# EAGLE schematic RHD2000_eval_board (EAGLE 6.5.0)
RHD2000 Evaluation Board

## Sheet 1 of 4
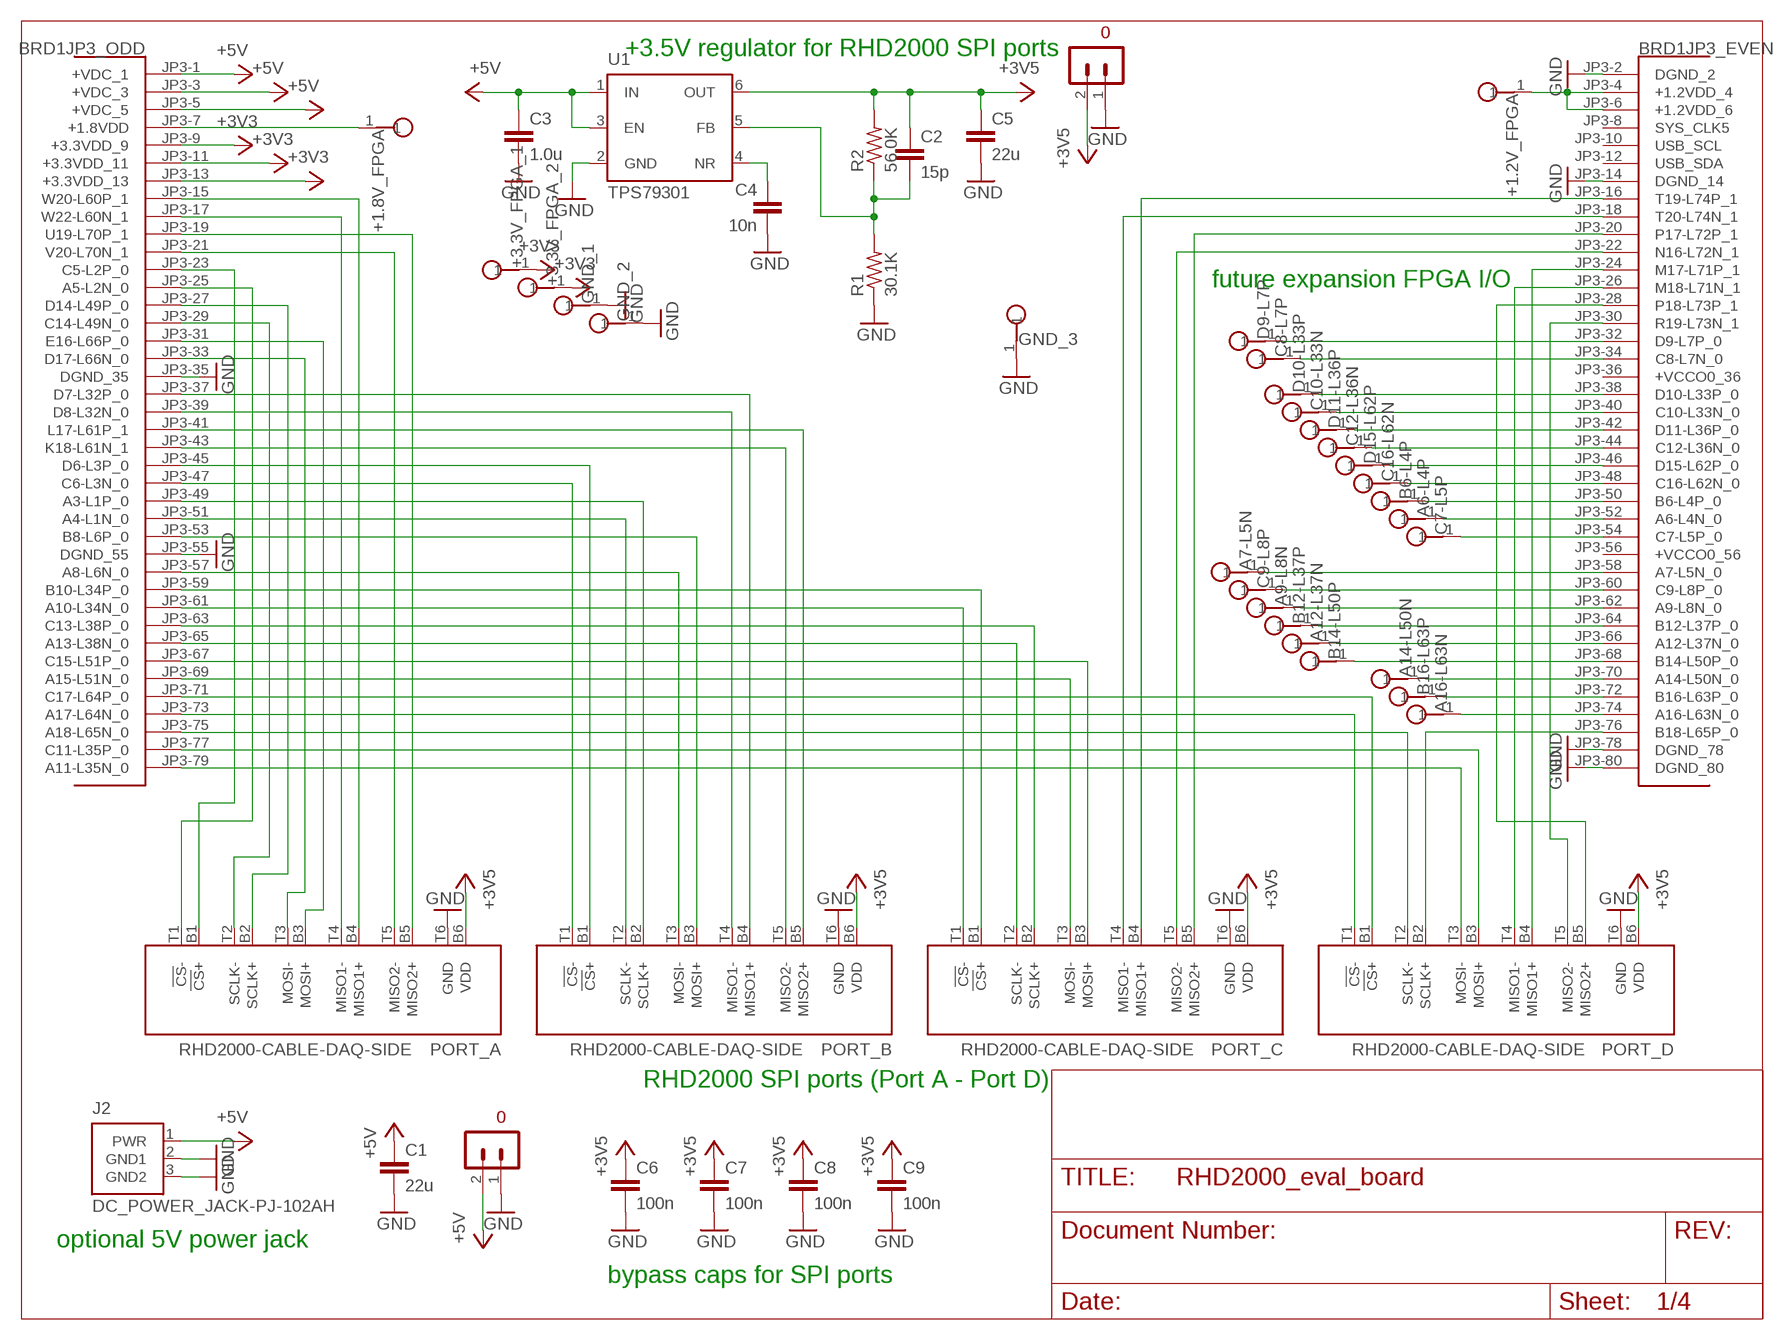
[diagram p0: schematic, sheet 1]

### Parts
+1.2V_FPGA  TESTPOINT  [TESTPOINT]
+1.8V_FPGA  TESTPOINT  [TESTPOINT]
+3.3V_FPGA_1  TESTPOINT  [TESTPOINT]
+3.3V_FPGA_2  TESTPOINT  [TESTPOINT]
A6-L4P  TESTPOINT  [TESTPOINT]
A7-L5N  TESTPOINT  [TESTPOINT]
A9-L8N  TESTPOINT  [TESTPOINT]
A12-L37N  TESTPOINT  [TESTPOINT]
A14-L50N  TESTPOINT  [TESTPOINT]
A16-L63N  TESTPOINT  [TESTPOINT]
B6-L4P  TESTPOINT  [TESTPOINT]
B12-L37P  TESTPOINT  [TESTPOINT]
B14-L50P  TESTPOINT  [TESTPOINT]
B16-L63P  TESTPOINT  [TESTPOINT]
BRD1  OPALKELLY_XEM6010  [OPALKELLY_XEM6010]
C1  22u  C_1206  [1206]
C2  15p  C_0603  [0603]
C3  1.0u  C_0805  [0805]
C4  10n  C_0603  [0603]
C5  22u  C_1206  [1206]
C6  100n  C_0603  [0603]
C7  100n  C_0603  [0603]
C7-L5P  TESTPOINT  [TESTPOINT]
C8  100n  C_0603  [0603]
C8-L7P  TESTPOINT  [TESTPOINT]
C9  100n  C_0603  [0603]
C9-L8P  TESTPOINT  [TESTPOINT]
C10-L33N  TESTPOINT  [TESTPOINT]
C12-L36N  TESTPOINT  [TESTPOINT]
C16-L62N  TESTPOINT  [TESTPOINT]
D9-L7P  TESTPOINT  [TESTPOINT]
D10-L33P  TESTPOINT  [TESTPOINT]
D11-L36P  TESTPOINT  [TESTPOINT]
D15-L62P  TESTPOINT  [TESTPOINT]
GND_1  TESTPOINT  [TESTPOINT]
GND_2  TESTPOINT  [TESTPOINT]
GND_3  TESTPOINT  [TESTPOINT]
J2  DC_POWER_JACK-PJ-102AH  [PJ-102AH]
PORT_A  RHD2000-CABLE-DAQ-SIDE  [OMNETICS_PZN-12-AA]
PORT_B  RHD2000-CABLE-DAQ-SIDE  [OMNETICS_PZN-12-AA]
PORT_C  RHD2000-CABLE-DAQ-SIDE  [OMNETICS_PZN-12-AA]
PORT_D  RHD2000-CABLE-DAQ-SIDE  [OMNETICS_PZN-12-AA]
R1  30.1K  R_0603  [0603]
R2  56.0K  R_0603  [0603]
S9  TERMINAL_BLOCK_2-3.5MM-5V  [TERMINAL_BLOCK_3.5MM_2_5V]
S10  TERMINAL_BLOCK_2-3.5MM-3.5V  [TERMINAL_BLOCK_3.5MM_2_3.5V]
U1  TPS79301  [SOT-23-6]

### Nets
+3V3 [power]: +3.3V_FPGA_1.1 +3.3V_FPGA_2.1 BRD1.JP3-9(JP3_ODD:+3.3VDD_9) BRD1.JP3-11(JP3_ODD:+3.3VDD_11) BRD1.JP3-13(JP3_ODD:+3.3VDD_13) ; also sheet 3
+3V5 [power]: C2.1 C5.1 C6.1 C7.1 C8.1 C9.1 PORT_A.B6(VDD) PORT_B.B6(VDD) PORT_C.B6(VDD) PORT_D.B6(VDD) R2.2 S10.2 U1.6(OUT)
+5V [power]: BRD1.JP3-1(JP3_ODD:+VDC_1) BRD1.JP3-3(JP3_ODD:+VDC_3) BRD1.JP3-5(JP3_ODD:+VDC_5) C1.1 C3.1 J2.1(PWR) S9.2 U1.1(IN) U1.3(EN) ; also sheet 2,4
GND [power]: BRD1.JP3-2(JP3_EVEN:DGND_2) BRD1.JP3-14(JP3_EVEN:DGND_14) BRD1.JP3-35(JP3_ODD:DGND_35) BRD1.JP3-55(JP3_ODD:DGND_55) BRD1.JP3-78(JP3_EVEN:DGND_78) BRD1.JP3-80(JP3_EVEN:DGND_80) C1.2 C3.2 C4.2 C5.2 C6.2 C7.2 C8.2 C9.2 GND_1.1 GND_2.1 GND_3.1 J2.2(GND1) J2.3(GND2) PORT_A.T6(GND) PORT_B.T6(GND) PORT_C.T6(GND) PORT_D.T6(GND) R1.1 S9.1 S10.1 U1.2(GND) ; also sheet 2,3,4
N$1: BRD1.JP3-15(JP3_ODD:W20-L60P_1) PORT_A.B4(MISO1+)
N$2: BRD1.JP3-17(JP3_ODD:W22-L60N_1) PORT_A.T4(MISO1-)
N$3: BRD1.JP3-19(JP3_ODD:U19-L70P_1) PORT_A.B5(MISO2+)
N$4: BRD1.JP3-21(JP3_ODD:V20-L70N_1) PORT_A.T5(MISO2-)
N$5: BRD1.JP3-23(JP3_ODD:C5-L2P_0) PORT_A.B1(!CS!+)
N$6: BRD1.JP3-25(JP3_ODD:A5-L2N_0) PORT_A.T1(!CS!-)
N$7: BRD1.JP3-27(JP3_ODD:D14-L49P_0) PORT_A.B2(SCLK+)
N$8: BRD1.JP3-29(JP3_ODD:C14-L49N_0) PORT_A.T2(SCLK-)
N$9: BRD1.JP3-31(JP3_ODD:E16-L66P_0) PORT_A.B3(MOSI+)
N$10: BRD1.JP3-33(JP3_ODD:D17-L66N_0) PORT_A.T3(MOSI-)
N$11: BRD1.JP3-37(JP3_ODD:D7-L32P_0) PORT_B.B4(MISO1+)
N$12: BRD1.JP3-39(JP3_ODD:D8-L32N_0) PORT_B.T4(MISO1-)
N$13: BRD1.JP3-41(JP3_ODD:L17-L61P_1) PORT_B.B5(MISO2+)
N$14: BRD1.JP3-43(JP3_ODD:K18-L61N_1) PORT_B.T5(MISO2-)
N$15: BRD1.JP3-45(JP3_ODD:D6-L3P_0) PORT_B.B1(!CS!+)
N$16: BRD1.JP3-47(JP3_ODD:C6-L3N_0) PORT_B.T1(!CS!-)
N$17: BRD1.JP3-49(JP3_ODD:A3-L1P_0) PORT_B.B2(SCLK+)
N$18: BRD1.JP3-51(JP3_ODD:A4-L1N_0) PORT_B.T2(SCLK-)
N$19: BRD1.JP3-53(JP3_ODD:B8-L6P_0) PORT_B.B3(MOSI+)
N$20: BRD1.JP3-57(JP3_ODD:A8-L6N_0) PORT_B.T3(MOSI-)
N$21: BRD1.JP3-59(JP3_ODD:B10-L34P_0) PORT_C.B1(!CS!+)
N$22: BRD1.JP3-61(JP3_ODD:A10-L34N_0) PORT_C.T1(!CS!-)
N$23: BRD1.JP3-63(JP3_ODD:C13-L38P_0) PORT_C.B2(SCLK+)
N$24: BRD1.JP3-65(JP3_ODD:A13-L38N_0) PORT_C.T2(SCLK-)
N$25: BRD1.JP3-67(JP3_ODD:C15-L51P_0) PORT_C.B3(MOSI+)
N$26: BRD1.JP3-69(JP3_ODD:A15-L51N_0) PORT_C.T3(MOSI-)
N$27: BRD1.JP3-71(JP3_ODD:C17-L64P_0) PORT_D.B1(!CS!+)
N$28: BRD1.JP3-73(JP3_ODD:A17-L64N_0) PORT_D.T1(!CS!-)
N$29: BRD1.JP3-75(JP3_ODD:A18-L65N_0) PORT_D.T2(SCLK-)
N$30: BRD1.JP3-77(JP3_ODD:C11-L35P_0) PORT_D.B3(MOSI+)
N$31: BRD1.JP3-79(JP3_ODD:A11-L35N_0) PORT_D.T3(MOSI-)
N$32: BRD1.JP3-76(JP3_EVEN:B18-L65P_0) PORT_D.B2(SCLK+)
N$33: BRD1.JP3-16(JP3_EVEN:T19-L74P_1) PORT_C.B4(MISO1+)
N$34: BRD1.JP3-18(JP3_EVEN:T20-L74N_1) PORT_C.T4(MISO1-)
N$35: BRD1.JP3-20(JP3_EVEN:P17-L72P_1) PORT_C.B5(MISO2+)
N$36: BRD1.JP3-22(JP3_EVEN:N16-L72N_1) PORT_C.T5(MISO2-)
N$37: BRD1.JP3-24(JP3_EVEN:M17-L71P_1) PORT_D.B4(MISO1+)
N$38: BRD1.JP3-26(JP3_EVEN:M18-L71N_1) PORT_D.T4(MISO1-)
N$39: BRD1.JP3-28(JP3_EVEN:P18-L73P_1) PORT_D.B5(MISO2+)
N$40: BRD1.JP3-30(JP3_EVEN:R19-L73N_1) PORT_D.T5(MISO2-)
N$143: C4.1 U1.4(NR)
N$144: C2.2 R1.2 R2.1 U1.5(FB)
N$173: BRD1.JP3-32(JP3_EVEN:D9-L7P_0) D9-L7P.1
N$174: BRD1.JP3-34(JP3_EVEN:C8-L7N_0) C8-L7P.1
N$175 [power]: +1.8V_FPGA.1 BRD1.JP3-7(JP3_ODD:+1.8VDD)
N$176: BRD1.JP3-38(JP3_EVEN:D10-L33P_0) D10-L33P.1
N$177: BRD1.JP3-40(JP3_EVEN:C10-L33N_0) C10-L33N.1
N$178: BRD1.JP3-42(JP3_EVEN:D11-L36P_0) D11-L36P.1
N$179: BRD1.JP3-44(JP3_EVEN:C12-L36N_0) C12-L36N.1
N$180: BRD1.JP3-46(JP3_EVEN:D15-L62P_0) D15-L62P.1
N$181: BRD1.JP3-48(JP3_EVEN:C16-L62N_0) C16-L62N.1
N$182: B6-L4P.1 BRD1.JP3-50(JP3_EVEN:B6-L4P_0)
N$183: A6-L4P.1 BRD1.JP3-52(JP3_EVEN:A6-L4N_0)
N$184: BRD1.JP3-54(JP3_EVEN:C7-L5P_0) C7-L5P.1
N$185 [power]: +1.2V_FPGA.1 BRD1.JP3-4(JP3_EVEN:+1.2VDD_4) BRD1.JP3-6(JP3_EVEN:+1.2VDD_6)
N$186: A7-L5N.1 BRD1.JP3-58(JP3_EVEN:A7-L5N_0)
N$187: BRD1.JP3-60(JP3_EVEN:C9-L8P_0) C9-L8P.1
N$188: A9-L8N.1 BRD1.JP3-62(JP3_EVEN:A9-L8N_0)
N$189: B12-L37P.1 BRD1.JP3-64(JP3_EVEN:B12-L37P_0)
N$190: A12-L37N.1 BRD1.JP3-66(JP3_EVEN:A12-L37N_0)
N$191: B14-L50P.1 BRD1.JP3-68(JP3_EVEN:B14-L50P_0)
N$192: A14-L50N.1 BRD1.JP3-70(JP3_EVEN:A14-L50N_0)
N$193: B16-L63P.1 BRD1.JP3-72(JP3_EVEN:B16-L63P_0)
N$194: A16-L63N.1 BRD1.JP3-74(JP3_EVEN:A16-L63N_0)
Unconnected: BRD1.JP3-8(JP3_EVEN:SYS_CLK5) BRD1.JP3-10(JP3_EVEN:USB_SCL) BRD1.JP3-12(JP3_EVEN:USB_SDA)

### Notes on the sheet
- +3.5V regulator for RHD2000 SPI ports
- future expansion FPGA I/O
- RHD2000 SPI ports (Port A - Port D)
- optional 5V power jack
- bypass caps for SPI ports

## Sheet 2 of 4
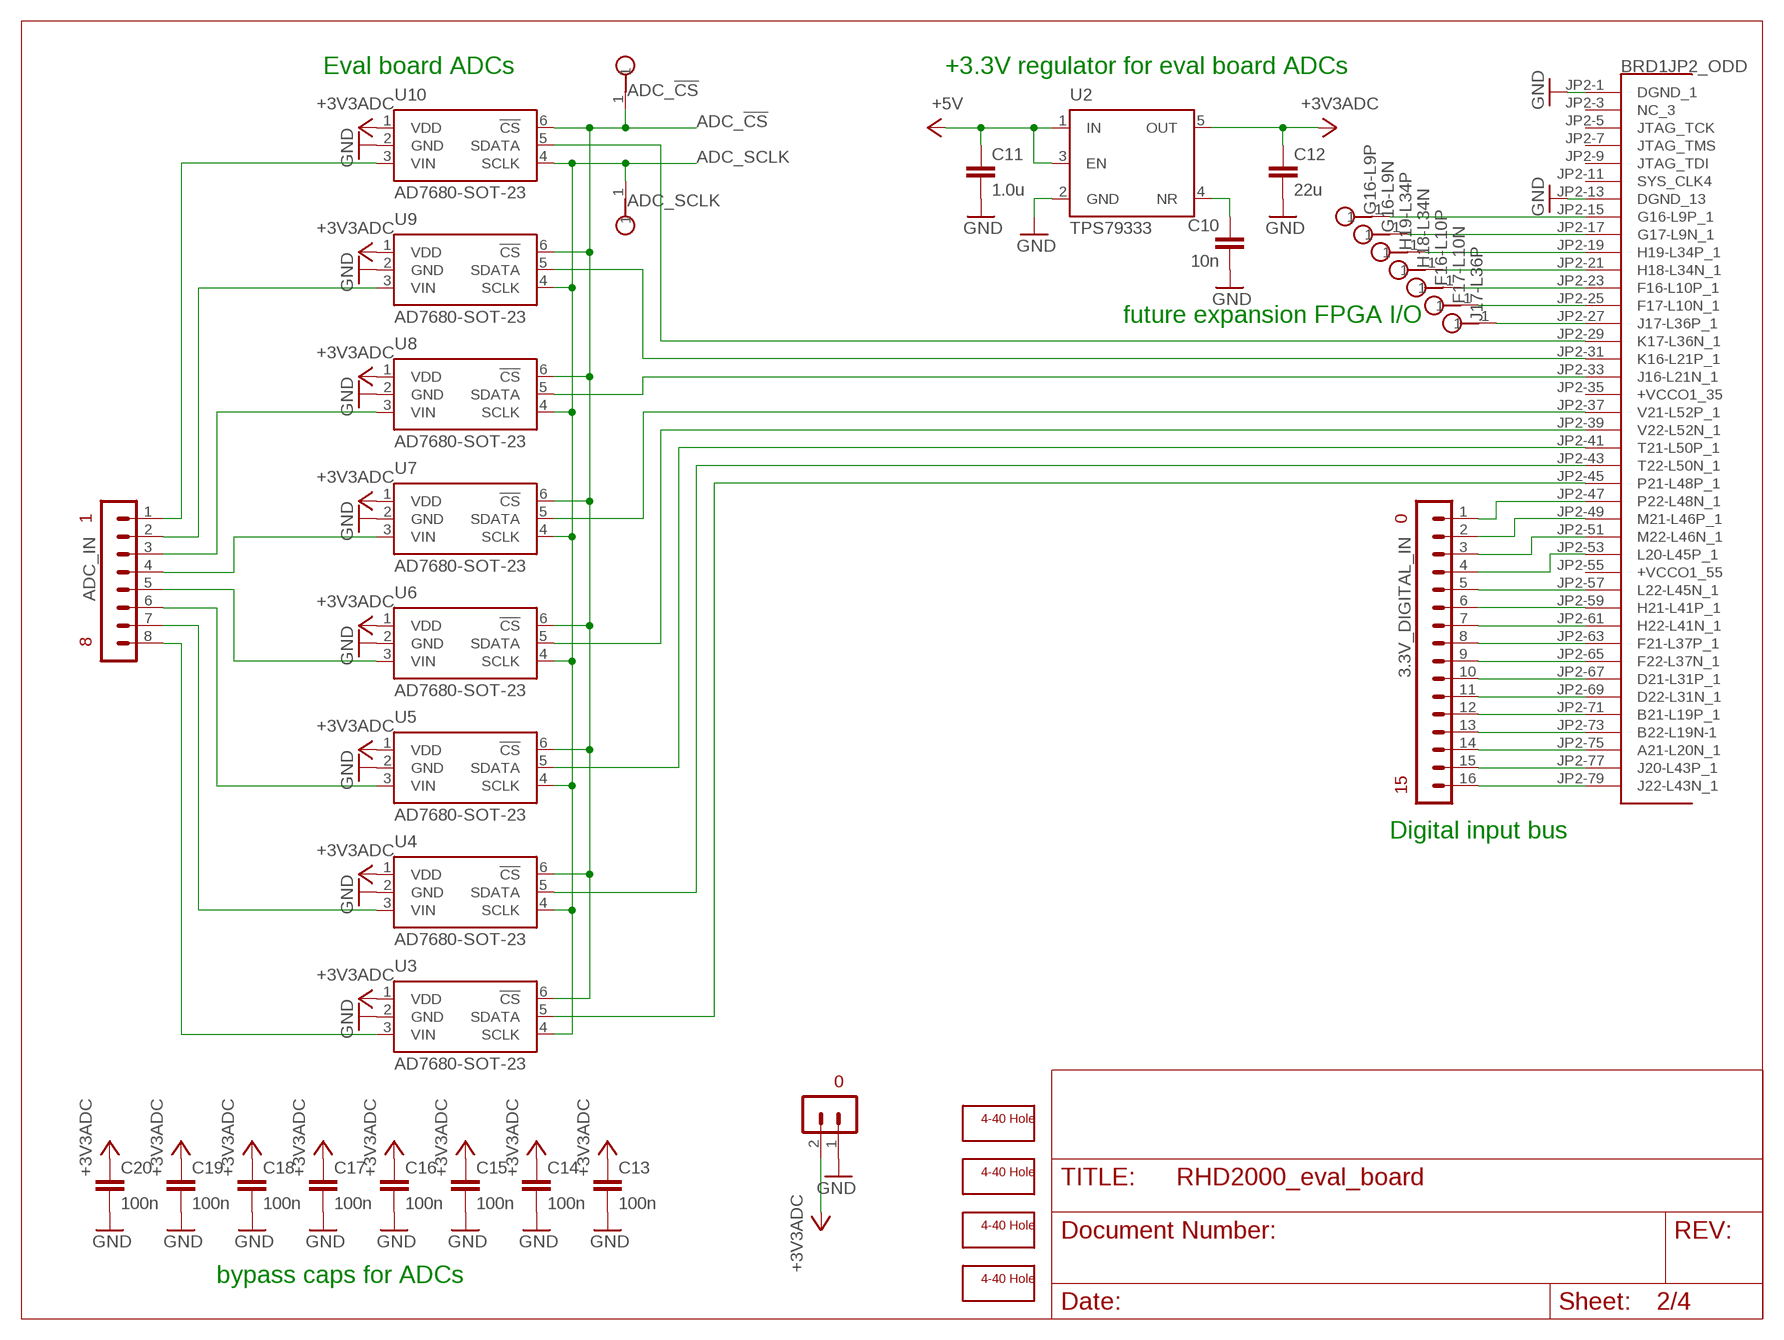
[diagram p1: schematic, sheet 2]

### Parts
3.3V_DIGITAL_IN  TERMINAL_BLOCK_16-3.5MM  [TERMINAL_BLOCK_3.5MM_16]
ADC_!CS!  TESTPOINT  [TESTPOINT]
ADC_IN  TERMINAL_BLOCK_8-3.5MM  [TERMINAL_BLOCK_3.5MM_8]
ADC_SCLK  TESTPOINT  [TESTPOINT]
C10  10n  C_0603  [0603]
C11  1.0u  C_0805  [0805]
C12  22u  C_1206  [1206]
C13  100n  C_0603  [0603]
C14  100n  C_0603  [0603]
C15  100n  C_0603  [0603]
C16  100n  C_0603  [0603]
C17  100n  C_0603  [0603]
C18  100n  C_0603  [0603]
C19  100n  C_0603  [0603]
C20  100n  C_0603  [0603]
F16-L10P  TESTPOINT  [TESTPOINT]
F17-L10N  TESTPOINT  [TESTPOINT]
G16-L9N  TESTPOINT  [TESTPOINT]
G16-L9P  TESTPOINT  [TESTPOINT]
H1  SCREW_HOLE_4-40  [SCREW_HOLE_4-40]
H2  SCREW_HOLE_4-40  [SCREW_HOLE_4-40]
H3  SCREW_HOLE_4-40  [SCREW_HOLE_4-40]
H4  SCREW_HOLE_4-40  [SCREW_HOLE_4-40]
H18-L34N  TESTPOINT  [TESTPOINT]
H19-L34P  TESTPOINT  [TESTPOINT]
J17-L36P  TESTPOINT  [TESTPOINT]
S2  TERMINAL_BLOCK_2-3.5MM-3.3V  [TERMINAL_BLOCK_3.5MM_2_3.3V]
U2  TPS79333  [SOT-23-5]
U3  AD7680-SOT-23  [SOT-23-RJ-6]
U4  AD7680-SOT-23  [SOT-23-RJ-6]
U5  AD7680-SOT-23  [SOT-23-RJ-6]
U6  AD7680-SOT-23  [SOT-23-RJ-6]
U7  AD7680-SOT-23  [SOT-23-RJ-6]
U8  AD7680-SOT-23  [SOT-23-RJ-6]
U9  AD7680-SOT-23  [SOT-23-RJ-6]
U10  AD7680-SOT-23  [SOT-23-RJ-6]

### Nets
+3V3ADC [power]: C12.1 C13.1 C14.1 C15.1 C16.1 C17.1 C18.1 C19.1 C20.1 S2.2 U2.5(OUT) U3.1(VDD) U4.1(VDD) U5.1(VDD) U6.1(VDD) U7.1(VDD) U8.1(VDD) U9.1(VDD) U10.1(VDD)
+5V [power]: C11.1 U2.1(IN) U2.3(EN) ; also sheet 1,4
ADC_!CS!: ADC_!CS!.1 U3.6(!CS!) U4.6(!CS!) U5.6(!CS!) U6.6(!CS!) U7.6(!CS!) U8.6(!CS!) U9.6(!CS!) U10.6(!CS!) ; also sheet 3
ADC_SCLK: ADC_SCLK.1 U3.4(SCLK) U4.4(SCLK) U5.4(SCLK) U6.4(SCLK) U7.4(SCLK) U8.4(SCLK) U9.4(SCLK) U10.4(SCLK) ; also sheet 3
GND [power]: BRD1.JP2-1(JP2_ODD:DGND_1) BRD1.JP2-13(JP2_ODD:DGND_13) C10.2 C11.2 C12.2 C13.2 C14.2 C15.2 C16.2 C17.2 C18.2 C19.2 C20.2 S2.1 U2.2(GND) U3.2(GND) U4.2(GND) U5.2(GND) U6.2(GND) U7.2(GND) U8.2(GND) U9.2(GND) U10.2(GND) ; also sheet 1,3,4
N$52: BRD1.JP2-29(JP2_ODD:K17-L36N_1) U10.5(SDATA)
N$54: BRD1.JP2-43(JP2_ODD:T22-L50N_1) U4.5(SDATA)
N$55: BRD1.JP2-31(JP2_ODD:K16-L21P_1) U9.5(SDATA)
N$56: BRD1.JP2-33(JP2_ODD:J16-L21N_1) U8.5(SDATA)
N$57: BRD1.JP2-37(JP2_ODD:V21-L52P_1) U7.5(SDATA)
N$58: BRD1.JP2-39(JP2_ODD:V22-L52N_1) U6.5(SDATA)
N$59: BRD1.JP2-41(JP2_ODD:T21-L50P_1) U5.5(SDATA)
N$60: BRD1.JP2-45(JP2_ODD:P21-L48P_1) U3.5(SDATA)
N$68: 3.3V_DIGITAL_IN.16 BRD1.JP2-79(JP2_ODD:J22-L43N_1)
N$69: 3.3V_DIGITAL_IN.15 BRD1.JP2-77(JP2_ODD:J20-L43P_1)
N$70: 3.3V_DIGITAL_IN.14 BRD1.JP2-75(JP2_ODD:A21-L20N_1)
N$71: 3.3V_DIGITAL_IN.13 BRD1.JP2-73(JP2_ODD:B22-L19N-1)
N$72: 3.3V_DIGITAL_IN.12 BRD1.JP2-71(JP2_ODD:B21-L19P_1)
N$73: 3.3V_DIGITAL_IN.11 BRD1.JP2-69(JP2_ODD:D22-L31N_1)
N$74: 3.3V_DIGITAL_IN.10 BRD1.JP2-67(JP2_ODD:D21-L31P_1)
N$75: 3.3V_DIGITAL_IN.9 BRD1.JP2-65(JP2_ODD:F22-L37N_1)
N$76: 3.3V_DIGITAL_IN.8 BRD1.JP2-63(JP2_ODD:F21-L37P_1)
N$77: 3.3V_DIGITAL_IN.7 BRD1.JP2-61(JP2_ODD:H22-L41N_1)
N$78: 3.3V_DIGITAL_IN.6 BRD1.JP2-59(JP2_ODD:H21-L41P_1)
N$79: 3.3V_DIGITAL_IN.5 BRD1.JP2-57(JP2_ODD:L22-L45N_1)
N$80: 3.3V_DIGITAL_IN.4 BRD1.JP2-53(JP2_ODD:L20-L45P_1)
N$81: 3.3V_DIGITAL_IN.3 BRD1.JP2-51(JP2_ODD:M22-L46N_1)
N$82: 3.3V_DIGITAL_IN.2 BRD1.JP2-49(JP2_ODD:M21-L46P_1)
N$83: 3.3V_DIGITAL_IN.1 BRD1.JP2-47(JP2_ODD:P22-L48N_1)
N$100: ADC_IN.1 U10.3(VIN)
N$101: ADC_IN.2 U9.3(VIN)
N$102: ADC_IN.3 U8.3(VIN)
N$103: ADC_IN.4 U7.3(VIN)
N$104: ADC_IN.5 U6.3(VIN)
N$105: ADC_IN.6 U5.3(VIN)
N$106: ADC_IN.7 U4.3(VIN)
N$107: ADC_IN.8 U3.3(VIN)
N$108: C10.1 U2.4(NR)
N$165: BRD1.JP2-15(JP2_ODD:G16-L9P_1) G16-L9P.1
N$166: BRD1.JP2-17(JP2_ODD:G17-L9N_1) G16-L9N.1
N$167: BRD1.JP2-19(JP2_ODD:H19-L34P_1) H19-L34P.1
N$168: BRD1.JP2-21(JP2_ODD:H18-L34N_1) H18-L34N.1
N$169: BRD1.JP2-23(JP2_ODD:F16-L10P_1) F16-L10P.1
N$170: BRD1.JP2-25(JP2_ODD:F17-L10N_1) F17-L10N.1
N$171: BRD1.JP2-27(JP2_ODD:J17-L36P_1) J17-L36P.1
Unconnected: BRD1.JP2-3(JP2_ODD:NC_3) BRD1.JP2-5(JP2_ODD:JTAG_TCK) BRD1.JP2-7(JP2_ODD:JTAG_TMS) BRD1.JP2-9(JP2_ODD:JTAG_TDI) BRD1.JP2-11(JP2_ODD:SYS_CLK4)

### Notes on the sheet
- Eval board ADCs | +3.3V regulator for eval board ADCs
- future expansion FPGA I/O
- Digital input bus
- bypass caps for ADCs

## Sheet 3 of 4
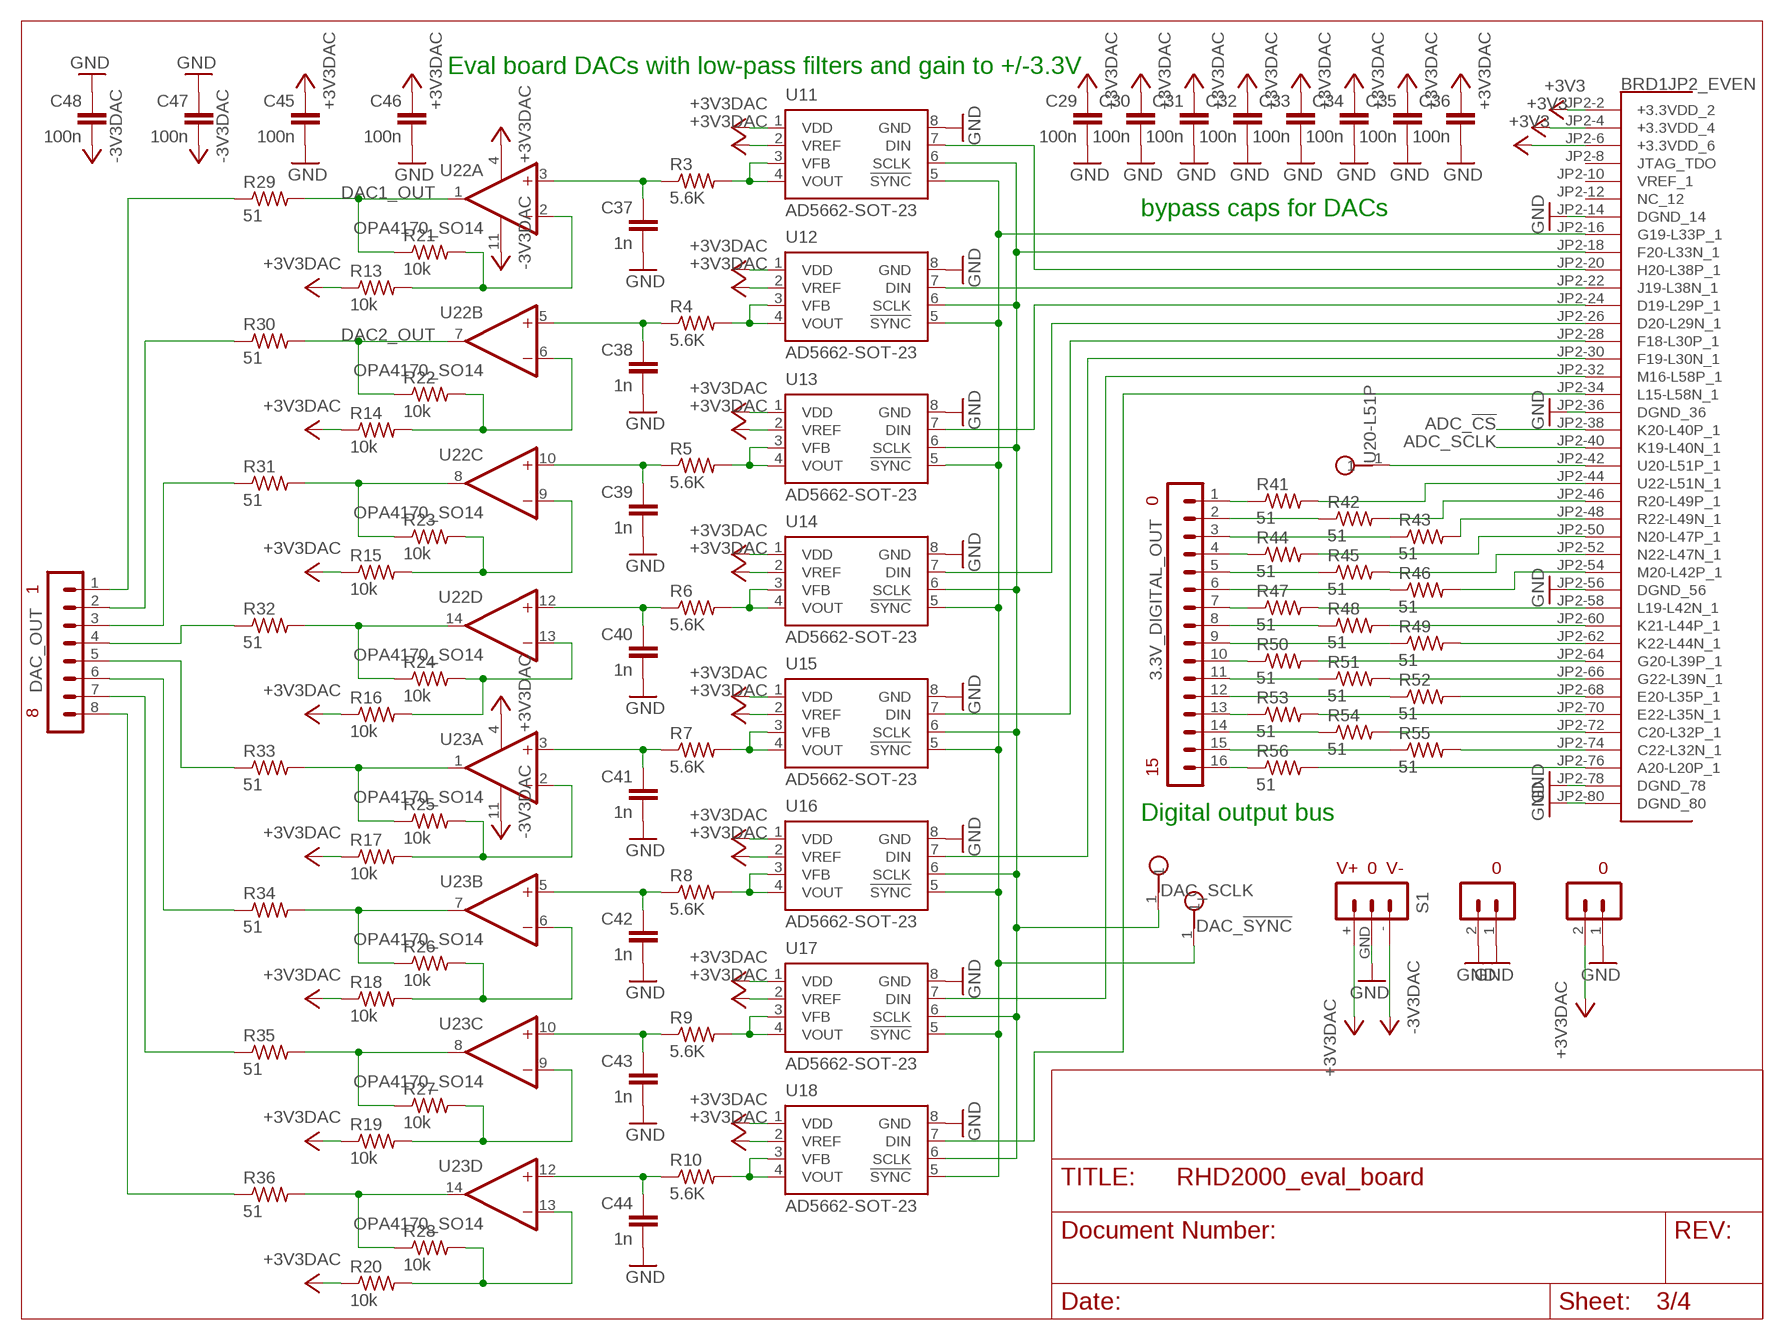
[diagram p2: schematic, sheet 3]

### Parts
3.3V_DIGITAL_OUT  TERMINAL_BLOCK_16-3.5MM  [TERMINAL_BLOCK_3.5MM_16]
C29  100n  C_0603  [0603]
C30  100n  C_0603  [0603]
C31  100n  C_0603  [0603]
C32  100n  C_0603  [0603]
C33  100n  C_0603  [0603]
C34  100n  C_0603  [0603]
C35  100n  C_0603  [0603]
C36  100n  C_0603  [0603]
C37  1n  C_0603  [0603]
C38  1n  C_0603  [0603]
C39  1n  C_0603  [0603]
C40  1n  C_0603  [0603]
C41  1n  C_0603  [0603]
C42  1n  C_0603  [0603]
C43  1n  C_0603  [0603]
C44  1n  C_0603  [0603]
C45  100n  C_0603  [0603]
C46  100n  C_0603  [0603]
C47  100n  C_0603  [0603]
C48  100n  C_0603  [0603]
DAC_!SYNC!  TESTPOINT  [TESTPOINT]
DAC_OUT  TERMINAL_BLOCK_8-3.5MM  [TERMINAL_BLOCK_3.5MM_8]
DAC_SCLK  TESTPOINT  [TESTPOINT]
R3  5.6K  R_0603  [0603]
R4  5.6K  R_0603  [0603]
R5  5.6K  R_0603  [0603]
R6  5.6K  R_0603  [0603]
R7  5.6K  R_0603  [0603]
R8  5.6K  R_0603  [0603]
R9  5.6K  R_0603  [0603]
R10  5.6K  R_0603  [0603]
R13  10k  R_0603  [0603]
R14  10k  R_0603  [0603]
R15  10k  R_0603  [0603]
R16  10k  R_0603  [0603]
R17  10k  R_0603  [0603]
R18  10k  R_0603  [0603]
R19  10k  R_0603  [0603]
R20  10k  R_0603  [0603]
R21  10k  R_0603  [0603]
R22  10k  R_0603  [0603]
R23  10k  R_0603  [0603]
R24  10k  R_0603  [0603]
R25  10k  R_0603  [0603]
R26  10k  R_0603  [0603]
R27  10k  R_0603  [0603]
R28  10k  R_0603  [0603]
R29  51  R_0603  [0603]
R30  51  R_0603  [0603]
R31  51  R_0603  [0603]
R32  51  R_0603  [0603]
R33  51  R_0603  [0603]
R34  51  R_0603  [0603]
R35  51  R_0603  [0603]
R36  51  R_0603  [0603]
R41  51  R_0603  [0603]
R42  51  R_0603  [0603]
R43  51  R_0603  [0603]
R44  51  R_0603  [0603]
R45  51  R_0603  [0603]
R46  51  R_0603  [0603]
R47  51  R_0603  [0603]
R48  51  R_0603  [0603]
R49  51  R_0603  [0603]
R50  51  R_0603  [0603]
R51  51  R_0603  [0603]
R52  51  R_0603  [0603]
R53  51  R_0603  [0603]
R54  51  R_0603  [0603]
R55  51  R_0603  [0603]
R56  51  R_0603  [0603]
S1  TERMINAL_BLOCK_3_+/-3.3V  [TERMINAL_BLOCK_3.5MM_3]
S6  TERMINAL_BLOCK_2-3.5MM-3.3V  [TERMINAL_BLOCK_3.5MM_2_3.3V]
S8  TERMINAL_BLOCK_2-3.5MM-GND  [TERMINAL_BLOCK_3.5MM_2_GND]
U11  AD5662-SOT-23  [SOT-23-RJ-8]
U12  AD5662-SOT-23  [SOT-23-RJ-8]
U13  AD5662-SOT-23  [SOT-23-RJ-8]
U14  AD5662-SOT-23  [SOT-23-RJ-8]
U15  AD5662-SOT-23  [SOT-23-RJ-8]
U16  AD5662-SOT-23  [SOT-23-RJ-8]
U17  AD5662-SOT-23  [SOT-23-RJ-8]
U18  AD5662-SOT-23  [SOT-23-RJ-8]
U20-L51P  TESTPOINT  [TESTPOINT]
U22  OPA4170_SO14  [SOIC-14]
U23  OPA4170_SO14  [SOIC-14]

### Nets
+3V3 [power]: BRD1.JP2-2(JP2_EVEN:+3.3VDD_2) BRD1.JP2-4(JP2_EVEN:+3.3VDD_4) BRD1.JP2-6(JP2_EVEN:+3.3VDD_6) ; also sheet 1
+3V3DAC [power]: C29.1 C30.1 C31.1 C32.1 C33.1 C34.1 C35.1 C36.1 C45.1 C46.1 R13.1 R14.1 R15.1 R16.1 R17.1 R18.1 R19.1 R20.1 S1.+ S6.2 U11.1(VDD) U11.2(VREF) U12.1(VDD) U12.2(VREF) U13.1(VDD) U13.2(VREF) U14.1(VDD) U14.2(VREF) U15.1(VDD) U15.2(VREF) U16.1(VDD) U16.2(VREF) U17.1(VDD) U17.2(VREF) U18.1(VDD) U18.2(VREF) U22.4(P:V+) U23.4(P:V+) ; also sheet 4
-3V3DAC [power]: C47.2 C48.2 S1.- U22.11(P:V-) U23.11(P:V-) ; also sheet 4
ADC_!CS!: BRD1.JP2-38(JP2_EVEN:K20-L40P_1) ; also sheet 2
ADC_SCLK: BRD1.JP2-40(JP2_EVEN:K19-L40N_1) ; also sheet 2
DAC1_OUT: R21.1 R29.2 U22.1(A:OUT) ; also sheet 4
DAC2_OUT: R22.1 R30.2 U22.7(B:OUT) ; also sheet 4
GND [power]: BRD1.JP2-14(JP2_EVEN:DGND_14) BRD1.JP2-36(JP2_EVEN:DGND_36) BRD1.JP2-56(JP2_EVEN:DGND_56) BRD1.JP2-78(JP2_EVEN:DGND_78) BRD1.JP2-80(JP2_EVEN:DGND_80) C29.2 C30.2 C31.2 C32.2 C33.2 C34.2 C35.2 C36.2 C37.2 C38.2 C39.2 C40.2 C41.2 C42.2 C43.2 C44.2 C45.2 C46.2 C47.1 C48.1 S1.GND S6.1 S8.1 S8.2 U11.8(GND) U12.8(GND) U13.8(GND) U14.8(GND) U15.8(GND) U16.8(GND) U17.8(GND) U18.8(GND) ; also sheet 1,2,4
N$41: BRD1.JP2-16(JP2_EVEN:G19-L33P_1) DAC_!SYNC!.1 U11.5(!SYNC!) U12.5(!SYNC!) U13.5(!SYNC!) U14.5(!SYNC!) U15.5(!SYNC!) U16.5(!SYNC!) U17.5(!SYNC!) U18.5(!SYNC!)
N$42: BRD1.JP2-18(JP2_EVEN:F20-L33N_1) DAC_SCLK.1 U11.6(SCLK) U12.6(SCLK) U13.6(SCLK) U14.6(SCLK) U15.6(SCLK) U16.6(SCLK) U17.6(SCLK) U18.6(SCLK)
N$43: BRD1.JP2-20(JP2_EVEN:H20-L38P_1) U11.7(DIN)
N$44: R13.2 R21.2 U22.2(A:-IN)
N$45: BRD1.JP2-22(JP2_EVEN:J19-L38N_1) U12.7(DIN)
N$46: BRD1.JP2-24(JP2_EVEN:D19-L29P_1) U13.7(DIN)
N$47: BRD1.JP2-26(JP2_EVEN:D20-L29N_1) U14.7(DIN)
N$48: BRD1.JP2-28(JP2_EVEN:F18-L30P_1) U15.7(DIN)
N$49: BRD1.JP2-30(JP2_EVEN:F19-L30N_1) U16.7(DIN)
N$50: BRD1.JP2-32(JP2_EVEN:M16-L58P_1) U17.7(DIN)
N$51: BRD1.JP2-34(JP2_EVEN:L15-L58N_1) U18.7(DIN)
N$53: DAC_OUT.2 R30.1
N$61: DAC_OUT.3 R31.1
N$62: DAC_OUT.4 R32.1
N$63: DAC_OUT.5 R33.1
N$64: DAC_OUT.6 R34.1
N$65: DAC_OUT.7 R35.1
N$66: DAC_OUT.8 R36.1
N$67: R3.2 U11.3(VFB) U11.4(VOUT)
N$84: BRD1.JP2-76(JP2_EVEN:A20-L20P_1) R56.2
N$85: BRD1.JP2-74(JP2_EVEN:C22-L32N_1) R55.2
N$86: BRD1.JP2-72(JP2_EVEN:C20-L32P_1) R54.2
N$87: BRD1.JP2-70(JP2_EVEN:E22-L35N_1) R53.2
N$88: BRD1.JP2-68(JP2_EVEN:E20-L35P_1) R52.2
N$89: BRD1.JP2-66(JP2_EVEN:G22-L39N_1) R51.2
N$90: BRD1.JP2-64(JP2_EVEN:G20-L39P_1) R50.2
N$91: BRD1.JP2-62(JP2_EVEN:K22-L44N_1) R49.2
N$92: BRD1.JP2-60(JP2_EVEN:K21-L44P_1) R48.2
N$93: BRD1.JP2-58(JP2_EVEN:L19-L42N_1) R47.2
N$94: BRD1.JP2-54(JP2_EVEN:M20-L42P_1) R46.2
N$95: BRD1.JP2-52(JP2_EVEN:N22-L47N_1) R45.2
N$96: BRD1.JP2-50(JP2_EVEN:N20-L47P_1) R44.2
N$97: BRD1.JP2-48(JP2_EVEN:R22-L49N_1) R43.2
N$98: BRD1.JP2-46(JP2_EVEN:R20-L49P_1) R42.2
N$99: BRD1.JP2-44(JP2_EVEN:U22-L51N_1) R41.2
N$109: C37.1 R3.1 U22.3(A:+IN)
N$111: R5.2 U13.3(VFB) U13.4(VOUT)
N$112: R6.2 U14.3(VFB) U14.4(VOUT)
N$113: DAC_OUT.1 R29.1
N$114: R4.2 U12.3(VFB) U12.4(VOUT)
N$115: R7.2 U15.3(VFB) U15.4(VOUT)
N$116: R8.2 U16.3(VFB) U16.4(VOUT)
N$117: R9.2 U17.3(VFB) U17.4(VOUT)
N$118: R10.2 U18.3(VFB) U18.4(VOUT)
N$119: R14.2 R22.2 U22.6(B:-IN)
N$120: C38.1 R4.1 U22.5(B:+IN)
N$122: C39.1 R5.1 U22.10(C:+IN)
N$123: R15.2 R23.2 U22.9(C:-IN)
N$124: C40.1 R6.1 U22.12(D:+IN)
N$125: R23.1 R31.2 U22.8(C:OUT)
N$126: C41.1 R7.1 U23.3(A:+IN)
N$128: C42.1 R8.1 U23.5(B:+IN)
N$129: R24.1 R32.2 U22.14(D:OUT)
N$130: C43.1 R9.1 U23.10(C:+IN)
N$131: R17.2 R25.2 U23.2(A:-IN)
N$132: C44.1 R10.1 U23.12(D:+IN)
N$133: R25.1 R33.2 U23.1(A:OUT)
N$134: R18.2 R26.2 U23.6(B:-IN)
N$135: R26.1 R34.2 U23.7(B:OUT)
N$136: R19.2 R27.2 U23.9(C:-IN)
N$137: R27.1 R35.2 U23.8(C:OUT)
N$138: R20.2 R28.2 U23.13(D:-IN)
N$139: R28.1 R36.2 U23.14(D:OUT)
N$142: R16.2 R24.2 U22.13(D:-IN)
N$147: 3.3V_DIGITAL_OUT.1 R41.1
N$148: 3.3V_DIGITAL_OUT.2 R42.1
N$149: 3.3V_DIGITAL_OUT.3 R43.1
N$151: 3.3V_DIGITAL_OUT.4 R44.1
N$152: 3.3V_DIGITAL_OUT.5 R45.1
N$153: 3.3V_DIGITAL_OUT.6 R46.1
N$154: 3.3V_DIGITAL_OUT.7 R47.1
N$155: 3.3V_DIGITAL_OUT.8 R48.1
N$156: 3.3V_DIGITAL_OUT.9 R49.1
N$157: 3.3V_DIGITAL_OUT.10 R50.1
N$158: 3.3V_DIGITAL_OUT.11 R51.1
N$159: 3.3V_DIGITAL_OUT.12 R52.1
N$160: 3.3V_DIGITAL_OUT.13 R53.1
N$161: 3.3V_DIGITAL_OUT.14 R54.1
N$162: 3.3V_DIGITAL_OUT.15 R55.1
N$163: 3.3V_DIGITAL_OUT.16 R56.1
N$172: BRD1.JP2-42(JP2_EVEN:U20-L51P_1) U20-L51P.1
Unconnected: BRD1.JP2-8(JP2_EVEN:JTAG_TDO) BRD1.JP2-10(JP2_EVEN:VREF_1) BRD1.JP2-12(JP2_EVEN:NC_12)

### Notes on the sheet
- Eval board DACs with low-pass filters and gain to +/-3.3V
- bypass caps for DACs
- Digital output bus

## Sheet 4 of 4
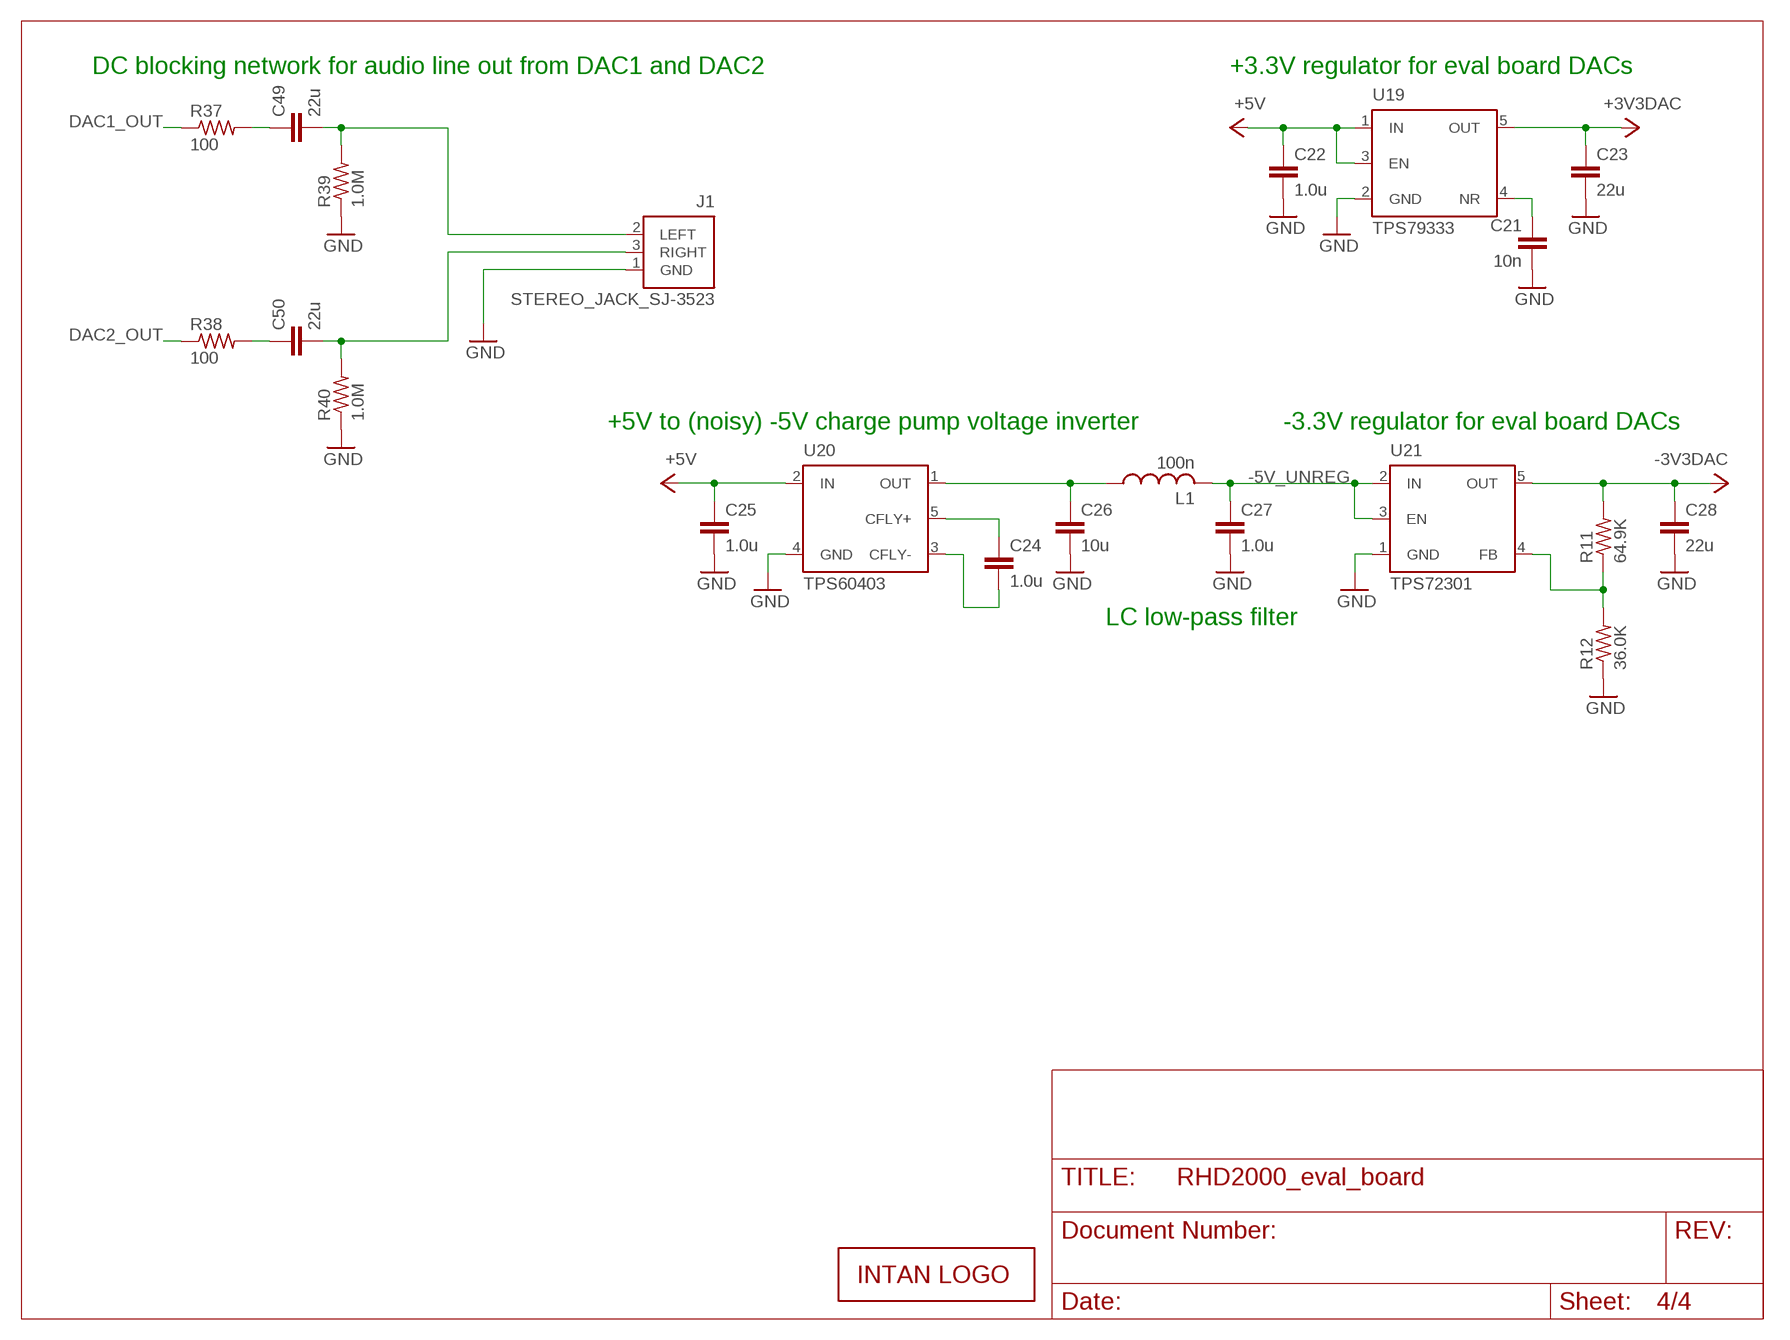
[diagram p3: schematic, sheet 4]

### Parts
C21  10n  C_0603  [0603]
C22  1.0u  C_0805  [0805]
C23  22u  C_1206  [1206]
C24  1.0u  C_0805  [0805]
C25  1.0u  C_0805  [0805]
C26  10u  C_1206  [1206]
C27  1.0u  C_0805  [0805]
C28  22u  C_1206  [1206]
C49  22u  C_1206  [1206]
C50  22u  C_1206  [1206]
J1  STEREO_JACK_SJ-3523  [SJ-3523]
L1  100n  L_0805  [0805]
LOGO1  INTAN_LOGO  [INTAN_LOGO]
R11  64.9K  R_0603  [0603]
R12  36.0K  R_0603  [0603]
R37  100  R_0603  [0603]
R38  100  R_0603  [0603]
R39  1.0M  R_0603  [0603]
R40  1.0M  R_0603  [0603]
U19  TPS79333  [SOT-23-5]
U20  TPS60403  [SOT-23-5]
U21  TPS72301  [SOT-23-5]

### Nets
+3V3DAC [power]: C23.1 U19.5(OUT) ; also sheet 3
+5V [power]: C22.1 C25.1 U19.1(IN) U19.3(EN) U20.2(IN) ; also sheet 1,2
-3V3DAC [power]: C28.1 R11.2 U21.5(OUT) ; also sheet 3
-5V_UNREG [power]: C27.1 L1.2 U21.2(IN) U21.3(EN)
DAC1_OUT: R37.1 ; also sheet 3
DAC2_OUT: R38.1 ; also sheet 3
GND [power]: C21.2 C22.2 C23.2 C25.2 C26.2 C27.2 C28.2 J1.1(GND) R12.1 R39.1 R40.1 U19.2(GND) U20.4(GND) U21.1(GND) ; also sheet 1,2,3
N$110: C49.1 R37.2
N$121: C50.1 R38.2
N$127: C50.2 J1.3(RIGHT) R40.2
N$140: C49.2 J1.2(LEFT) R39.2
N$141: C21.1 U19.4(NR)
N$145 [power]: C24.1 U20.5(CFLY+)
N$146 [power]: C24.2 U20.3(CFLY-)
N$150: R11.1 R12.2 U21.4(FB)
N$164 [power]: C26.1 L1.1 U20.1(OUT)

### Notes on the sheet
- DC blocking network for audio line out from DAC1 and DAC2 | +3.3V regulator for eval board DACs
- +5V to (noisy) -5V charge pump voltage inverter | -3.3V regulator for eval board DACs
- LC low-pass filter

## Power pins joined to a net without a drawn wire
+VCCO0_36: BRD1.JP3-36(JP3_EVEN:+VCCO0_36)
+VCCO0_56: BRD1.JP3-56(JP3_EVEN:+VCCO0_56)
+VCCO1_35: BRD1.JP2-35(JP2_ODD:+VCCO1_35)
+VCCO1_55: BRD1.JP2-55(JP2_ODD:+VCCO1_55)

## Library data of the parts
3.3V_DIGITAL_IN 3.3V_DIGITAL_OUT = RHD2000_eval_board:TERMINAL_BLOCK_16: 16-point terminal block
+1.2V_FPGA +1.8V_FPGA +3.3V_FPGA_1 +3.3V_FPGA_2 A6-L4P A7-L5N A9-L8N A12-L37N A14-L50N A16-L63N ADC_!CS! ADC_SCLK B6-L4P B12-L37P B14-L50P B16-L63P C7-L5P C8-L7P C9-L8P C10-L33N C12-L36N C16-L62N D9-L7P D10-L33P D11-L36P D15-L62P DAC_!SYNC! DAC_SCLK F16-L10P F17-L10N G16-L9N G16-L9P GND_1-GND_3 H18-L34N H19-L34P J17-L36P U20-L51P = RHD2000_eval_board:TESTPOINT: PCB Test Point
ADC_IN DAC_OUT = RHD2000_eval_board:TERMINAL_BLOCK_8: 8-point terminal block
BRD1 = RHD2000_eval_board:OPALKELLY_XEM6010: Opal Kelly XEM6010 USB/FPGA module
C1-C50 = RHD2000_eval_board:C: Capacitor
H1-H4 = RHD2000_eval_board:SCREW_HOLE_4-40: Mounting hole
J1 = RHD2000_eval_board:STEREO_JACK: CUI Inc. SJ-3523 stereo audio jack
J2 = RHD2000_eval_board:DC_POWER_JACK: DC Power Jack
L1 = RHD2000_eval_board:L: Inductor
LOGO1 = RHD2000_eval_board:INTAN_LOGO
PORT_A PORT_B PORT_C PORT_D = RHD2000_eval_board:RHD2000-CABLE-DAQ-SIDE: Omnetics PZN-12-AA RHD2000 socket - DAQ side
R1-R56 = RHD2000_eval_board:R: Resistor
S1 = RHD2000_eval_board:TERMINAL_BLOCK_3: 3-point terminal block
S2 S6 S8-S10 = RHD2000_eval_board:TERMINAL_BLOCK_2: 2-point terminal block
U1 = RHD2000_eval_board:TPS79301: Texas Instruments TPS79301 adjustable regulator
U2 U19 = RHD2000_eval_board:TPS79333: Texas Instruments TPS79333 3.3V LDO regulator
U3-U10 = RHD2000_eval_board:AD7680: Analog Devices AD7680 16-bit ADC
U11-U18 = RHD2000_eval_board:AD5662: Analog Devices AD5662 16-bit DAC
U20 = RHD2000_eval_board:TPS60403: Texas Instruments TPS60403 voltage inverter
U21 = RHD2000_eval_board:TPS72301: Texas Instruments TPS62301 adjustable negative regulator
U22 U23 = RHD2000_eval_board:OPA4170: TI OPA4170 quad op amp

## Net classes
1 power: width 0.381 mm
